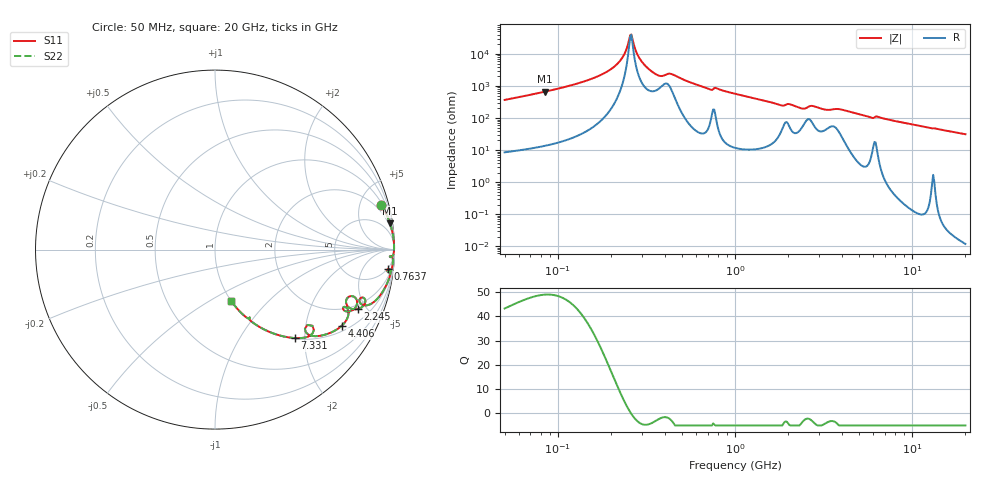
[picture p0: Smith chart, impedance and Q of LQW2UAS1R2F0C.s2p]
!Murata Part Number: LQW2UAS1R2F0C
!These Parameters are Measured in Series Mode Connection
!  o--[Z]--o
!Port1  Port2
!  o-------o
!Freq. Start=50[MHz] Stop=20[GHz], 401[Steps]
# Hz S RI R 50
!Freq.(Hz) S11(Real) S11(Imag) S21(Real) S21(Imag) S12(Real) S12(Imag) S22(Real) S22(Imag)
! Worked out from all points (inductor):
!   401 points, 50 MHz to 20 GHz, reference 50 ohm
!   read as one part in series: L = 1.12 uH near 51.52 MHz
!   highest Q = 48.9 at 84.46 MHz (marker M1), where L = 1.25 uH
!   self-resonance near 255.9 MHz
!   S11 on the Smith chart (normalised r, x): 50 MHz: 1.17, +7.36; 763.7 MHz: 5, -17; 2.245 GHz: 1.70, -4.37; 4.406 GHz: 1.20, -3.18; 7.331 GHz: 1.01, -1.79; 20 GHz: 1.00, -0.63
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5e7  0.9262 0.2501  0.0738 -0.2501  0.0738 -0.2501  0.9262 0.2501
8.445984e7  0.975 0.1463  0.025 -0.1463  0.025 -0.1463  0.975 0.1463
1.364002e8  0.9924 0.0754  0.00759 -0.0754  0.00759 -0.0754  0.9924 0.0754
1.759554e8  0.9964 0.0441  0.00363 -0.0441  0.00363 -0.0441  0.9964 0.0441
2.106029e8  0.9977 0.0234  0.00232 -0.0234  0.00232 -0.0234  0.9977 0.0234
2.33884e8  0.9979 0.0115  0.00211 -0.0115  0.00211 -0.0115  0.9979 0.0115
2.520729e8  0.9977 0.00295  0.00226 -0.00295  0.00226 -0.00295  0.9977 0.00295
2.597386e8  0.9976 -0.000522  0.00241 0.000522  0.00241 0.000522  0.9976 -0.000522
2.799383e8  0.9969 -0.00938  0.00309 0.00938  0.00309 0.00938  0.9969 -0.00938
2.972233e8  0.9959 -0.0167  0.0041 0.0167  0.0041 0.0167  0.9959 -0.0167
3.300798e8  0.9921 -0.0302  0.00787 0.0302  0.00787 0.0302  0.9921 -0.0302
3.721004e8  0.9797 -0.0422  0.0203 0.0422  0.0203 0.0422  0.9797 -0.0422
4.322267e8  0.9837 -0.0376  0.0163 0.0376  0.0163 0.0376  0.9837 -0.0376
7.08568e8  0.9783 -0.1187  0.0217 0.1187  0.0217 0.1187  0.9783 -0.1187
7.636728e8  0.9638 -0.1072  0.0362 0.1072  0.0362 0.1072  0.9638 -0.1072
1e9  0.9671 -0.1685  0.0329 0.1685  0.0329 0.1685  0.9671 -0.1685
2.245319e9  0.7953 -0.3312  0.2047 0.3312  0.2047 0.3312  0.7953 -0.3312
2.728004e9  0.7893 -0.2797  0.2107 0.2797  0.2107 0.2797  0.7893 -0.2797
4.405649e9  0.7053 -0.425  0.2947 0.425  0.2947 0.425  0.7053 -0.425
7.331367e9  0.4454 -0.4929  0.5546 0.4929  0.5546 0.4929  0.4454 -0.4929
7.442007e9  0.4364 -0.4923  0.5636 0.4923  0.5636 0.4923  0.4364 -0.4923
2e10  0.0891 -0.2847  0.9109 0.2847  0.9109 0.2847  0.0891 -0.2847
